(* Logix 5000 AddOnInstructionDefinition export AMCI_SD4840E2_Run_Blend_Move; software revision 20.03 *)

ADD_ON_INSTRUCTION AMCI_SD4840E2_Run_Blend_Move   (* revision 5.0, vendor AMCI, ExecuteEnableInFalse *)
// Revision note:
// Version 5.0 added the (hidden) ability to program the motor current and unlatched the error bit if the rung goes false.
VAR_INPUT
   Axis_Status_Bits : INT; {required}
   Type_0_for_standard_1_for_indexed : BOOL;
   Direction_0_for_CW_1_for_CCW : BOOL; {required}
   motor_current : INT;
END_VAR
VAR_IN_OUT
   AMCI_SD4840E2_output_data : _000A:SD4840E2_4342D302:O:0; {required}
END_VAR
VAR_OUTPUT
   EN : BOOL; {access Read Only, visible}
   ER : BOOL; {access Read Only, visible}
END_VAR
VAR
   command_data_block : INT[10];
        [0]   // Command Bits MSW
        [1]   // Command Bits LSW
        [2]   // Upper Target Position
        [3]   // Lower Target Position
        [4]   // Upper Programmed Speed
        [5]   // Lower Programmed Speed
END_VAR

ROUTINE EnableInFalse   (* ladder *)
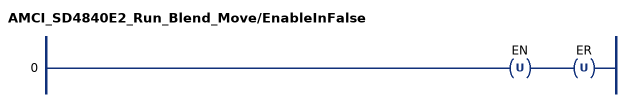
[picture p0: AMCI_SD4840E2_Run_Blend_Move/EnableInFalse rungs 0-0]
   0: OTU(EN)OTU(ER);
END_ROUTINE

ROUTINE Logic   (* ladder *)
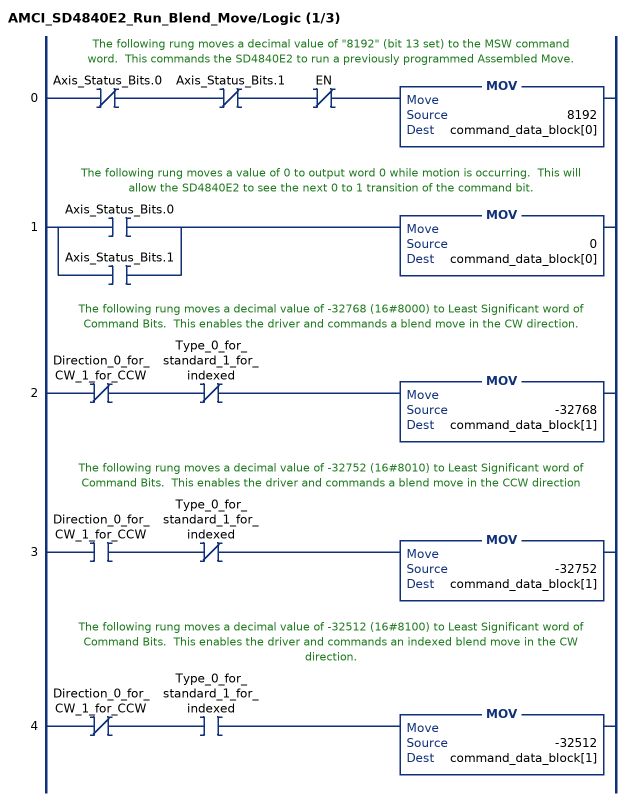
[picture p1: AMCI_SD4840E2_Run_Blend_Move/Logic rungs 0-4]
   // The following rung moves a decimal value of "8192" (bit 13 set) to the MSW command word.  This commands the SD4840E2 to run a previously programmed Assembled Move.
   0: XIO(Axis_Status_Bits.0)XIO(Axis_Status_Bits.1)XIO(EN)MOV(8192,command_data_block[0]);
   // The following rung moves a value of 0 to output word 0 while motion is occurring.  This will allow the SD4840E2 to see the next 0 to 1 transition of the command bit.
   1: [XIC(Axis_Status_Bits.0) ,XIC(Axis_Status_Bits.1) ]MOV(0,command_data_block[0]);
   // The following rung moves a decimal value of -32768 (16#8000) to Least Significant word of Command Bits.  This enables the driver and commands a blend move in the CW direction.
   2: XIO(Direction_0_for_CW_1_for_CCW)XIO(Type_0_for_standard_1_for_indexed)MOV(-32768,command_data_block[1]);
   // The following rung moves a decimal value of -32752 (16#8010) to Least Significant word of Command Bits.  This enables the driver and commands a blend move in the CCW direction
   3: XIC(Direction_0_for_CW_1_for_CCW)XIO(Type_0_for_standard_1_for_indexed)MOV(-32752,command_data_block[1]);
   // The following rung moves a decimal value of -32512 (16#8100) to Least Significant word of Command Bits.  This enables the driver and commands an indexed blend move in the CW direction.
   4: XIO(Direction_0_for_CW_1_for_CCW)XIC(Type_0_for_standard_1_for_indexed)MOV(-32512,command_data_block[1]);
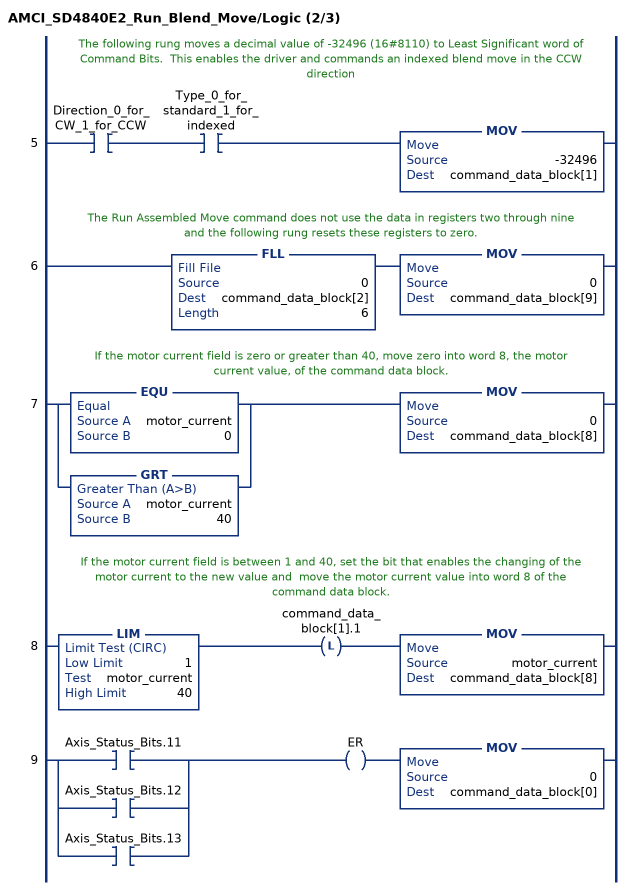
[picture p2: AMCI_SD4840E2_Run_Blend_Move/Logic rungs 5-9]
   // The following rung moves a decimal value of -32496 (16#8110) to Least Significant word of Command Bits.  This enables the driver and commands an indexed blend move in the CCW direction
   5: XIC(Direction_0_for_CW_1_for_CCW)XIC(Type_0_for_standard_1_for_indexed)MOV(-32496,command_data_block[1]);
   // The Run Assembled Move command does not use the data in registers two through nine and the following rung resets these registers to zero.
   6: FLL(0,command_data_block[2],6)MOV(0,command_data_block[9]);
   // If the motor current field is zero or greater than 40, move zero into word 8, the motor current value, of the command data block.
   7: [EQU(motor_current,0) ,GRT(motor_current,40) ]MOV(0,command_data_block[8]);
   // If the motor current field is between 1 and 40, set the bit that enables the changing of the motor current to the new value and  move the motor current value into word 8 of the command data block.
   8: LIM(1,motor_current,40)OTL(command_data_block[1].1)MOV(motor_current,command_data_block[8]);
   9: [XIC(Axis_Status_Bits.11) ,XIC(Axis_Status_Bits.12) ,XIC(Axis_Status_Bits.13) ]OTE(ER)MOV(0,command_data_block[0]);
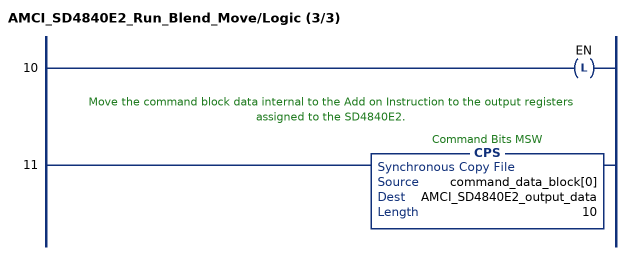
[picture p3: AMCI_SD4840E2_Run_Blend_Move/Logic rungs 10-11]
   10: OTL(EN);
   // Move the command block data internal to the Add on Instruction to the output registers assigned to the SD4840E2.
   11: CPS(command_data_block[0],AMCI_SD4840E2_output_data,10);
END_ROUTINE
END_ADD_ON_INSTRUCTION
